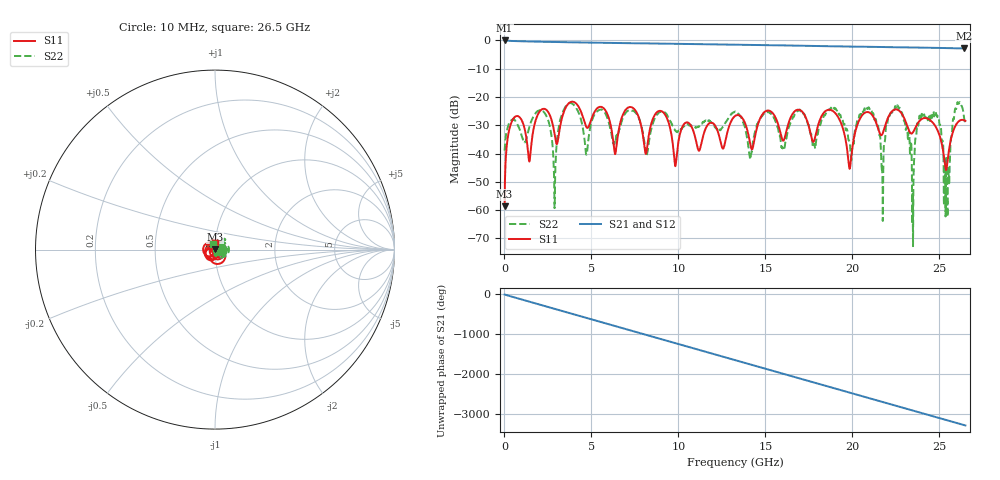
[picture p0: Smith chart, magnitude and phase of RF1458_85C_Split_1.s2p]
!Keysight Technologies,N5245B,MY55451909,A.13.80.08
!Automatic Fixture Removal (AFR)
!Date: Thursday, August 27, 2020, 03:55:00
!S2P File: Measurements: S11,S21,S12,S22:
# MHz S  RI  R 50
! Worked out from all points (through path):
!   2650 points, 10 MHz to 26.5 GHz, reference 50 ohm
!   highest |S21| = -0.01 dB at 10 MHz (marker M1); lowest = -2.8 dB at 26.43 GHz (marker M2)
!   group delay of S21, straight-line fit = 344 ps
!   lowest |S11| = -58.7 dB at 10 MHz (marker M3), VSWR 1.00, Z = 50 + j0.115 ohm
!   |S11| at or under -10 dB: start of sweep to end of sweep
!   |S22| runs from -72.8 to -21.8 dB; largest |S21 - S12| = 1.4e-15
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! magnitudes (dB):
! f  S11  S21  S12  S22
! 10 MHz  -58.7  0.0  0.0  -39.0
! 590 MHz  -27.1  -0.2  -0.2  -28.2
! 1.43 GHz  -42.8  -0.4  -0.4  -30.7
! 2.26 GHz  -24.2  -0.5  -0.5  -25.3
! 2.88 GHz  -33.0  -0.5  -0.5  -59.3
! 3.51 GHz  -23.9  -0.6  -0.6  -23.4
! 4.43 GHz  -25.7  -0.7  -0.7  -28.7
! 8.13 GHz  -40.2  -1.0  -1.0  -39.8
! 8.84 GHz  -25.1  -1.1  -1.1  -25.8
! 9.83 GHz  -44.5  -1.2  -1.2  -31.9
! 13.26 GHz  -26.7  -1.5  -1.5  -25.2
! 17.67 GHz  -34.8  -1.9  -1.9  -34.6
! 18.86 GHz  -24.9  -2.1  -2.1  -24.0
! 19.85 GHz  -45.4  -2.2  -2.2  -36.0
! 20.89 GHz  -25.3  -2.3  -2.3  -24.0
! 21.75 GHz  -32.8  -2.3  -2.3  -63.9
! 22.09 GHz  -26.8  -2.4  -2.4  -27.2
! 23.44 GHz  -32.8  -2.5  -2.5  -65.0
! 24.85 GHz  -31.2  -2.6  -2.6  -26.4
! 25.39 GHz  -45.8  -2.7  -2.7  -43.7
! 26.43 GHz  -28.2  -2.8  -2.8  -27.6
! 26.5 GHz  -28.5  -2.8  -2.8  -29.7
